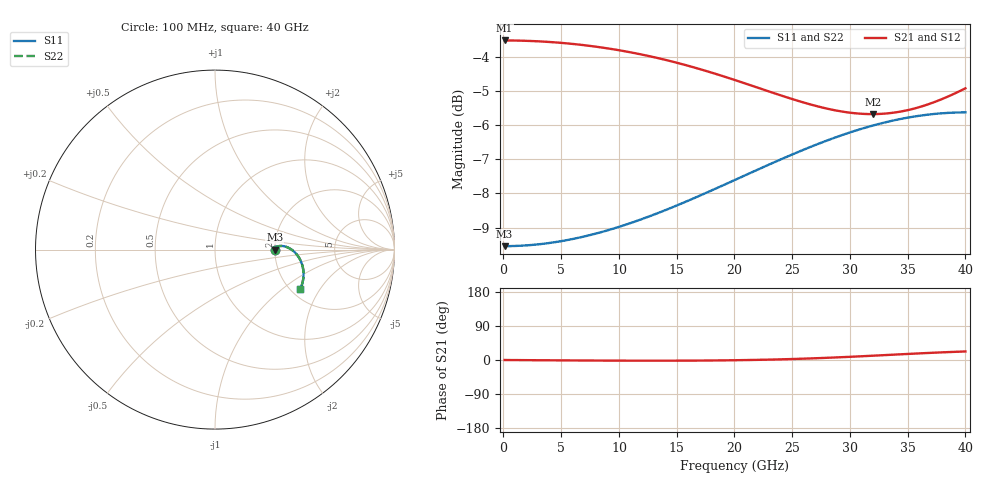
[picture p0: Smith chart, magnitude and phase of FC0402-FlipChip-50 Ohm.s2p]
!Vishay Thin-Film
!FC Family
!Case Size 0402
!Assembly Style Flip-Chip
!10/21/2015
!thinfilm@vishay.com
# GHz S MA R 50
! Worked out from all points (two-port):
!   101 points, 100 MHz to 40 GHz, reference 50 ohm
!   highest |S21| = -3.52 dB at 100 MHz (marker M1); lowest = -5.7 dB at 32.02 GHz (marker M2)
!   |S21| within 3 dB of the highest: start of sweep to end of sweep
!   lowest |S11| = -9.5 dB at 100 MHz (marker M3), VSWR 2.00, Z = 100 + j0.0534 ohm
!   |S11| at or under -10 dB: nowhere
!   |S22| runs from -9.5 to -5.6 dB; largest |S21 - S12| = 0
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0.1  0.3333 0.0  0.6667 -0.0  0.6667 -0.0  0.3333 0.0
3.292  0.3358 1.3  0.6643 -0.7  0.6643 -0.7  0.3358 1.3
4.888  0.3388 1.9  0.6615 -1.0  0.6615 -1.0  0.3388 1.9
6.883  0.3441 2.5  0.6564 -1.3  0.6564 -1.3  0.3441 2.5
10.075  0.3561 3.1  0.6447 -1.7  0.6447 -1.7  0.3561 3.1
13.666  0.3743 3.1  0.6265 -1.8  0.6265 -1.8  0.3743 3.1
16.858  0.3942 2.3  0.6063 -1.5  0.6063 -1.5  0.3942 2.3
18.454  0.4052 1.7  0.5951 -1.1  0.5951 -1.1  0.4052 1.7
20.05  0.4167 0.8  0.5834 -0.6  0.5834 -0.6  0.4167 0.8
22.045  0.4316 -0.5  0.5684 0.4  0.5684 0.4  0.4316 -0.5
23.641  0.4437 -1.8  0.5567 1.5  0.5567 1.5  0.4437 -1.8
25.237  0.4557 -3.4  0.5457 2.8  0.5457 2.8  0.4557 -3.4
26.833  0.4675 -5.1  0.5359 4.4  0.5359 4.4  0.4675 -5.1
28.03  0.4759 -6.5  0.5298 5.8  0.5298 5.8  0.4759 -6.5
29.626  0.4866 -8.5  0.5237 7.9  0.5237 7.9  0.4866 -8.5
30.823  0.494 -10.1  0.521 9.6  0.521 9.6  0.494 -10.1
32.02  0.5007 -11.8  0.5202 11.4  0.5202 11.4  0.5007 -11.8
33.616  0.5085 -14.2  0.5222 13.8  0.5222 13.8  0.5085 -14.2
35.212  0.5147 -16.7  0.5281 16.3  0.5281 16.3  0.5147 -16.7
36.808  0.5193 -19.3  0.5378 18.6  0.5378 18.6  0.5193 -19.3
38.404  0.5222 -21.9  0.5511 20.7  0.5511 20.7  0.5222 -21.9
40  0.5232 -24.5  0.5674 22.5  0.5674 22.5  0.5232 -24.5
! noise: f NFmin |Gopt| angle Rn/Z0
0.1  0  1  -8.538e-07  1
4.489  9.643e-16  1  -8.538e-07  1.019
8.878  -3.857e-15  1  -8.538e-07  1.078
13.27  1.929e-15  1  1.919e-15  1.179
17.66  -9.643e-16  1  6.117e-15  1.328
22.05  9.643e-16  1  -1.207e-06  1.518
26.43  -1.446e-15  1  -1.608e-15  1.707
30.82  1.634e-07  1  -4.923e-15  1.785
35.21  1.497e-07  1  -8.716e-15  1.635
40  9.643e-16  1  -5.9e-15  1.256
